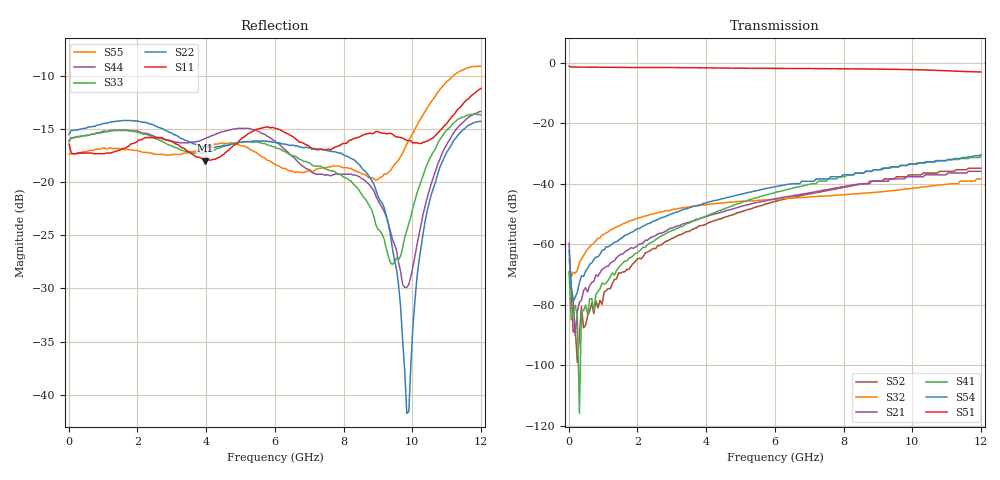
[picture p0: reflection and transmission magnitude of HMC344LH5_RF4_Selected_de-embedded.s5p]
! Hittite Microwave Corporation
! 20 Alpha Road
! Chelmsford, MA 01824
! Tel: 978-250-3343
! Fax: 978-250-3373
! Device: HMC344LH5, DC-12 GHz GaAs MMIC SP4T Non-Reflective Switch in Hermetic Leadless SMT Package
! Misc: Data was de-embedded to package pins.
!  Port 1 = RFC
!  Port 2 = RF1
!  Port 3 = RF2
!  Port 4 = RF3
!  Port 5 = RF4
!  RF4 selected, Vctl= 0/-5 V
!  Data reformated to new Touchstone file format - Tue Jan 09 16:01:08 2007
# MHz S DB R 50
! 5 Port Network Data
! freq  dbS11  angS11  dbS12  angS12  dbS13  angS13  dbS14  angS14
!  dbS15  angS15
!  dbS21  angS21  dbS22  angS22  dbS23  angS23
!  dbS24  angS24  dbS25  angS25
!  dbS31  angS31  dbS32  angS32
!  dbS33  angS33  dbS34  angS34  dbS35  angS35
!  dbS41  angS41
!  dbS42  angS42  dbS43  angS43  dbS44  angS44  dbS45  angS45
!  dbS51  angS51  dbS52  angS52  dbS53  angS53  dbS54  angS54
!  dbS55  angS55
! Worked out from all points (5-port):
!   201 points, 10 MHz to 12 GHz, reference 50 ohm
!   strongest paths, dB at 10 MHz, 3.007 GHz, 6.005 GHz, 9.002 GHz, 12 GHz:
!     S51: -1.2, -1.6, -1.9, -2.2, -3.1
!     S54: -62.2, -49.9, -41.0, -35.4, -30.5
!     S41: -69.4, -55.4, -42.9, -35.4, -31.1
!     S21: -59.7, -54.7, -45.0, -39.2, -35.9
!     S32: -65.2, -48.6, -45.1, -42.8, -38.4
!     S52: -69.1, -58.1, -45.8, -39.2, -34.9
!   lowest |S11| = -18.0 dB at 3.967 GHz (marker M1), VSWR 1.29, Z = 42.7 - j9.18 ohm
!   |S11| at or under -10 dB: start of sweep to end of sweep
